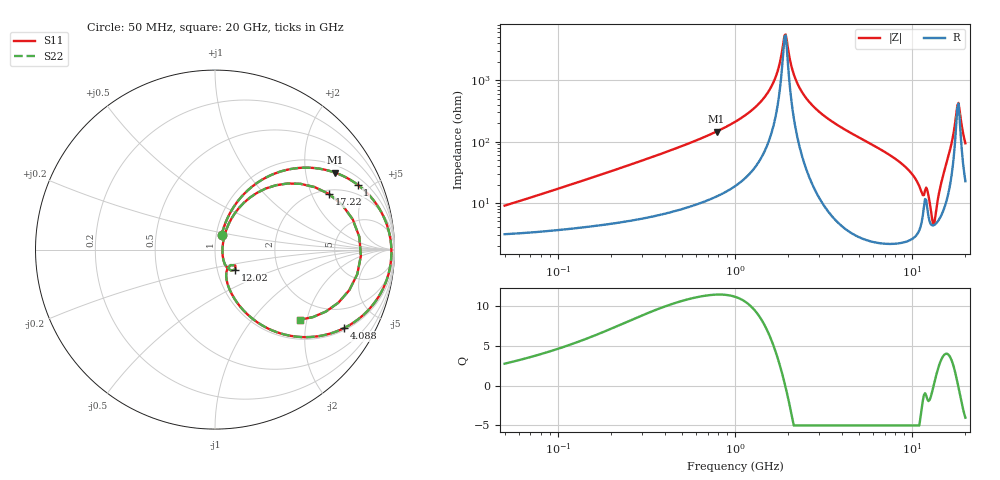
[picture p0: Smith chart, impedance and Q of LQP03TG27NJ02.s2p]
!Murata Part Number: LQP03TG27NJ02
!These Parameters are Measured in Series Mode Connection
!  o--[Z]--o
!Port1  Port2
!  o-------o
!Freq. Start=50[MHz] Stop=20[GHz], 401[Steps]
# Hz S RI R 50
!Freq.(Hz) S11(Real) S11(Imag) S21(Real) S21(Imag) S12(Real) S12(Imag) S22(Real) S22(Imag)
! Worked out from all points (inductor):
!   401 points, 50 MHz to 20 GHz, reference 50 ohm
!   read as one part in series: L = 26.8 nH near 56.37 MHz
!   highest Q = 11.4 at 786.9 MHz (marker M1), where L = 29.4 nH
!   self-resonance near 1.904 GHz
!   S11 on the Smith chart (normalised r, x): 50 MHz: 1.06, +0.17; 1 GHz: 1.38, +4.18; 4.088 GHz: 1.08, -3.26; 12.02 GHz: 1.22, -0.28; 17.22 GHz: 2.18, +2.70; 20 GHz: 1.45, -1.82
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5e7  0.0366 0.0795  0.9634 -0.0795  0.9634 -0.0795  0.0366 0.0795
1.364002e8  0.0813 0.1988  0.9187 -0.1988  0.9187 -0.1988  0.0813 0.1988
3.721004e8  0.2934 0.4064  0.7066 -0.4064  0.7066 -0.4064  0.2934 0.4064
7.868965e8  0.6669 0.4295  0.3331 -0.4295  0.3331 -0.4295  0.6669 0.4295
1e9  0.7942 0.3619  0.2058 -0.3619  0.2058 -0.3619  0.7942 0.3619
1.544007e9  0.9564 0.142  0.0436 -0.142  0.0436 -0.142  0.9564 0.142
1.714689e9  0.9745 0.0752  0.0255 -0.0752  0.0255 -0.0752  0.9745 0.0752
1.875929e9  0.9821 0.0157  0.0179 -0.0157  0.0179 -0.0157  0.9821 0.0157
1.932977e9  0.9829 -0.00439  0.0171 0.00439  0.0171 0.00439  0.9829 -0.00439
2.211938e9  0.9757 -0.0956  0.0243 0.0956  0.0243 0.0956  0.9757 -0.0956
2.728004e9  0.9284 -0.2332  0.0716 0.2332  0.0716 0.2332  0.9284 -0.2332
4.087748e9  0.7214 -0.4362  0.2786 0.4362  0.2786 0.4362  0.7214 -0.4362
7.442007e9  0.2779 -0.4306  0.7221 0.4306  0.7221 0.4306  0.2779 -0.4306
9.457416e9  0.1277 -0.3016  0.8723 0.3016  0.8723 0.3016  0.1277 -0.3016
1.201863e10  0.114 -0.1112  0.886 0.1112  0.886 0.1112  0.114 -0.1112
1.295331e10  0.0428 -0.0339  0.9572 0.0339  0.9572 0.0339  0.0428 -0.0339
1.334722e10  0.0422 0.0138  0.9578 -0.0138  0.9578 -0.0138  0.0422 0.0138
1.527346e10  0.1605 0.2607  0.8395 -0.2607  0.8395 -0.2607  0.1605 0.2607
1.646126e10  0.4037 0.3684  0.5963 -0.3684  0.5963 -0.3684  0.4037 0.3684
1.721783e10  0.6343 0.3104  0.3657 -0.3104  0.3657 -0.3104  0.6343 0.3104
1.828096e10  0.8128 -0.0345  0.1872 0.0345  0.1872 0.0345  0.8128 -0.0345
2e10  0.4747 -0.3905  0.5253 0.3905  0.5253 0.3905  0.4747 -0.3905
